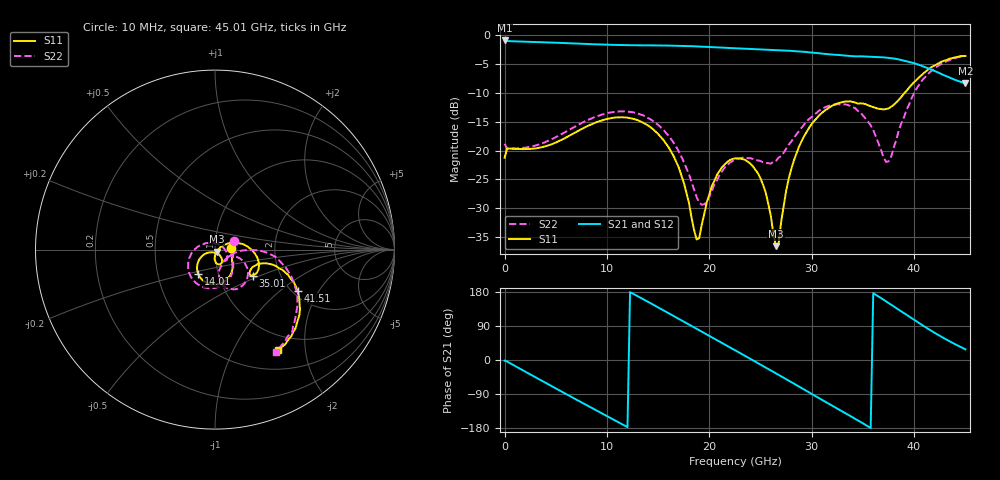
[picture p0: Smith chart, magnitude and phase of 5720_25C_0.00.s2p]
! Device:  ADRF5720
! Description: 0.5dB LSB GaAs MMIC 6-bit Digital Attenuator
! Frequency:  0.000009 -  40 GHz
! Ports:
!	RF1	= Port 1
!	RF2	= Port 2
! Vdd:  3.3 Volt
! Vss:  -3.3 Volt
! Control:  0/3.3 Volt
! State:  0.00 dB attenuation
! Data:  The device was measured using G-S-G Probes on a matrix board.
!  Data was collected using an calibrated 4 port network analyzer.
!  The reference plane for this measurement is at the launchers.
! Note:  Analog Devices supplies this data as a sample of measured data
!  for this product.  Your particular data for this product may vary.
!  Data was taken at 25 degrees C.
!  Analog Devices reserves the right to change this data at anytime.
# GHZ S DB R 45.0
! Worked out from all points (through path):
!   181 points, 10 MHz to 45.01 GHz, reference 45 ohm
!   highest |S21| = -0.92 dB at 10 MHz (marker M1); lowest = -8.4 dB at 45.01 GHz (marker M2)
!   group delay of S21, straight-line fit = 42.6 ps
!   lowest |S11| = -36.5 dB at 26.51 GHz (marker M3), VSWR 1.03, Z = 45.9 - j0.974 ohm
!   |S11| at or under -10 dB: start of sweep to 39.07 GHz
!   |S22| runs from -29.4 to -3.6 dB; largest |S21 - S12| = 0.0011
!   S11 on the Smith chart (normalised r, x): 10 MHz: 1.19, +0.02; 14.01 GHz: 0.80, -0.22; 35.01 GHz: 1.45, -0.45; 41.51 GHz: 2.13, -1.34; 45.01 GHz: 0.77, -1.53
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0.01  -21.23 4.2  -0.92 -1.7  -0.92 -1.8  -18.81 25.2
2.01  -19.74 -17.7  -1.13 -30.6  -1.14 -30.6  -19.49 -17.7
4.26  -19.10 -31.2  -1.27 -63.9  -1.27 -63.9  -18.31 -33.6
7.76  -16.04 -54.4  -1.50 -115.4  -1.50 -115.4  -15.01 -62.1
11.01  -14.24 -88.5  -1.70 -162.6  -1.70 -162.6  -13.23 -98.5
14.01  -15.64 -124.4  -1.77 153.6  -1.77 153.6  -14.31 -138.8
15.26  -17.62 -138.7  -1.79 135.0  -1.79 135.0  -15.95 -157.4
17.01  -22.88 -155.3  -1.85 108.7  -1.85 108.8  -20.10 171.4
18.76  -35.38 -110.5  -1.95 82.2  -1.95 82.3  -28.04 112.3
19.51  -30.95 -56.7  -2.01 70.9  -2.01 70.9  -29.30 58.9
20.76  -24.17 -52.9  -2.12 52.0  -2.12 52.1  -25.12 -1.2
22.76  -21.32 -71.7  -2.29 21.9  -2.29 22.0  -21.42 -36.3
25.01  -24.85 -91.3  -2.47 -12.1  -2.47 -12.0  -21.80 -46.8
26.51  -36.55 -45.5  -2.58 -35.1  -2.58 -35.1  -21.77 -31.0
28.26  -21.71 25.0  -2.76 -62.3  -2.76 -62.3  -17.79 -18.6
30.26  -14.82 5.7  -3.06 -93.6  -3.06 -93.6  -13.73 -29.6
35.01  -11.85 -34.4  -3.68 -167.2  -3.68 -167.1  -13.94 -77.5
37.26  -12.81 -26.9  -3.89 154.8  -3.90 154.9  -21.95 -50.1
37.76  -12.38 -21.9  -3.99 146.1  -4.00 146.2  -21.08 -19.9
39.76  -8.59 -16.2  -4.74 110.3  -4.74 110.4  -10.91 -3.0
41.51  -5.77 -26.6  -5.86 79.9  -5.85 80.0  -6.47 -22.5
45.01  -3.62 -57.7  -8.37 28.1  -8.37 28.1  -3.58 -59.0
